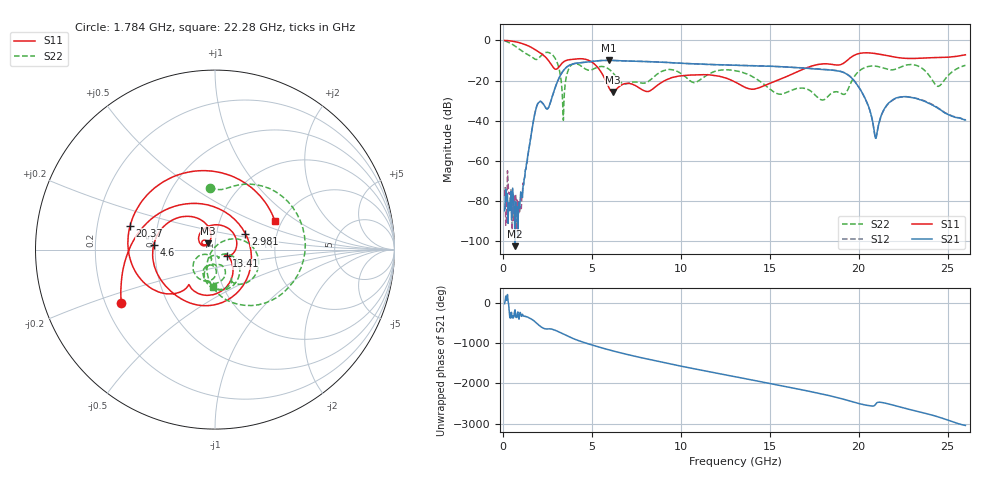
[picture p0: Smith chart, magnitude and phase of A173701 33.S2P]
!  2-Port S-parameters saved by WinCal
! VAR MeasName=S-Parameters (CALIBRATED_DATA) read from VNA (N5245A)
! VAR MeasDate=2017-6-7 10:30:39
! VAR NAME=A173701 33
! VAR FILENAME=A173701 33.S2P
! VAR DATE=2017-6-7 10:30:39
! VAR PHYS_PORTS=1,2
# Hz S DB R 50
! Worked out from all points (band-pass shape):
!   801 points, 100 MHz to 26 GHz, reference 50 ohm
!   highest |S21| = -9.93 dB at 5.96 GHz (marker M1); lowest = -102.6 dB at 682.8 MHz (marker M2)
!   |S21| within 3 dB of the highest: 3.642 GHz to 15.21 GHz (11.56 GHz wide, 123 % of centre)
!   lowest |S11| = -25.7 dB at 6.186 GHz (marker M3), VSWR 1.11, Z = 46.2 + j3.29 ohm
!   |S11| at or under -10 dB: 2.563 GHz to 3.554 GHz (991.8 MHz wide, 32.4 % of centre); 4.842 GHz to 19.35 GHz (14.51 GHz wide, 120 % of centre)
!   |S22| runs from -39.8 to -0.2 dB; largest |S21 - S12| = 0.0042
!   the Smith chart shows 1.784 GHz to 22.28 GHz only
!   S11 on the Smith chart (normalised r, x): 1.784 GHz: 0.27, -0.25; 2.981 GHz: 1.38, +0.26; 4.6 GHz: 0.49, +0.03; 13.41 GHz: 1.14, -0.08; 20.37 GHz: 0.35, +0.12; 22.28 GHz: 1.84, +0.67
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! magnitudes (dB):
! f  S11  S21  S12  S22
! 100 MHz  0.0  -84.9  -77.5  -0.2
! 682.8 MHz  -0.6  -102.6  -78.0  -2.8
! 1.039 GHz  -1.4  -76.5  -83.8  -5.0
! 1.784 GHz  -4.4  -37.1  -37.0  -9.2
! 2.981 GHz  -14.4  -22.5  -22.5  -9.6
! 3.402 GHz  -10.8  -15.1  -15.1  -39.8
! 3.791 GHz  -9.6  -12.2  -12.2  -12.9
! 4.438 GHz  -9.1  -11.0  -11.0  -13.0
! 4.6 GHz  -9.3  -10.9  -10.9  -14.0
! 5.96 GHz  -23.5  -9.9  -9.9  -14.3
! 6.186 GHz  -25.7  -10.0  -10.0  -16.1
! 8.744 GHz  -22.0  -10.8  -10.8  -16.4
! 13.05 GHz  -20.7  -12.4  -12.4  -15.1
! 13.41 GHz  -22.4  -12.5  -12.4  -15.7
! 17.39 GHz  -12.7  -14.1  -14.0  -25.9
! 19.2 GHz  -11.0  -16.1  -16.1  -26.9
! 20.37 GHz  -6.2  -29.0  -29.0  -13.5
! 20.95 GHz  -6.6  -48.8  -49.0  -12.8
! 21.69 GHz  -7.8  -31.1  -31.4  -14.5
! 22.28 GHz  -8.6  -28.3  -28.4  -13.6
! 24.48 GHz  -8.5  -34.0  -33.7  -22.9
! 26 GHz  -7.2  -39.6  -39.6  -12.4
